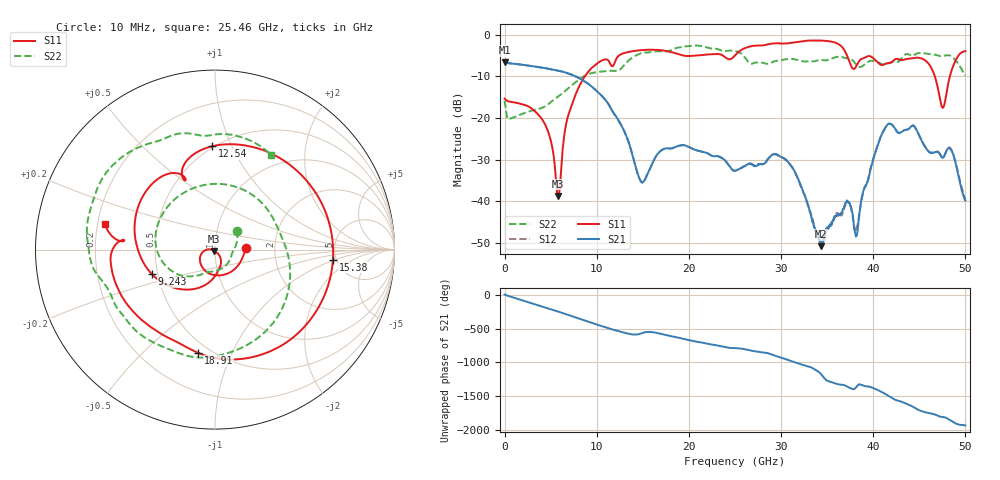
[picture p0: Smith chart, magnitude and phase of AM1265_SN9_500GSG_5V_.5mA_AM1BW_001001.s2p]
!Keysight Technologies,N5245B,MY58422270,A.16.20.02
!Date: Thursday, March 05, 2026 00:32:22
!Correction: S11(C  2-Port  )
!S21(C  2-Port  )
!S12(C  2-Port  )
!S22(C  2-Port  )
!S2P File: Measurements: S11, S21, S12, S22:
# Hz S  dB  R 50
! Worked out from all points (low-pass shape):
!   3201 points, 10 MHz to 50 GHz, reference 50 ohm
!   highest |S21| = -6.62 dB at 10 MHz (marker M1); lowest = -50.7 dB at 34.36 GHz (marker M2)
!   |S21| within 3 dB of the highest: start of sweep to 7.338 GHz
!   lowest |S11| = -38.7 dB at 5.821 GHz (marker M3), VSWR 1.02, Z = 49.4 - j0.975 ohm
!   |S11| at or under -10 dB: start of sweep to 8.715 GHz; 46.69 GHz to 48.31 GHz (1.624 GHz wide, 3.42 % of centre)
!   |S22| runs from -20.3 to -2.6 dB; largest |S21 - S12| = 0.002
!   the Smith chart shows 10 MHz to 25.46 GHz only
!   S11 on the Smith chart (normalised r, x): 10 MHz: 1.41, +0.03; 9.243 GHz: 0.46, -0.15; 12.54 GHz: 0.49, +0.84; 15.38 GHz: 4.68, -0.93; 18.91 GHz: 0.43, -0.75; 25.46 GHz: 0.23, +0.11
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1e7  -15.34 3.3  -6.62 2.8  -6.65 3.0  -15.82 40.3
2.306416e9  -16.94 -91.6  -7.30 -97.9  -7.30 -97.9  -18.69 -83.1
4.649697e9  -22.77 -167.1  -8.11 162.3  -8.11 162.3  -16.82 -114.4
5.821338e9  -38.67 -122.1  -8.62 111.1  -8.61 111.2  -14.80 -126.6
6.743028e9  -20.80 -70.1  -9.16 69.5  -9.15 69.5  -13.18 -137.0
8.352081e9  -11.32 -124.8  -10.73 -4.6  -10.72 -4.6  -10.33 -168.9
9.242528e9  -8.47 -158.7  -12.03 -45.7  -12.02 -45.6  -9.32 165.2
1.253874e10  -4.79 91.7  -21.19 175.4  -21.21 175.5  -8.33 7.4
1.538192e10  -3.62 -4.9  -34.04 168.8  -34.02 168.9  -4.28 -112.0
1.667854e10  -3.65 -43.5  -28.40 150.5  -28.40 150.7  -4.02 -142.2
1.891247e10  -4.68 -99.2  -26.65 84.5  -26.62 84.9  -3.07 -179.3
2.5005e10  -4.96 173.5  -32.67 -68.3  -32.58 -68.9  -3.91 71.2
2.545803e10  -4.00 166.9  -32.23 -73.9  -32.21 -73.9  -4.24 59.6
3.039455e10  -2.11 82.1  -29.77 133.2  -29.89 133.1  -5.92 -46.2
3.334708e10  -1.39 35.5  -44.21 0.4  -43.73 4.5  -6.39 -127.8
3.43625e10  -1.39 17.9  -50.72 -97.6  -50.31 -105.6  -6.05 -149.4
3.717444e10  -5.07 -41.1  -39.93 82.6  -40.08 83.7  -5.68 156.4
3.818986e10  -7.43 -22.4  -48.11 79.5  -46.62 74.7  -7.25 139.2
4.167354e10  -6.81 -54.5  -21.37 -57.2  -21.36 -57.5  -6.82 114.0
4.509473e10  -5.59 -102.3  -24.67 87.6  -24.65 88.6  -4.37 75.1
4.770358e10  -16.86 70.6  -29.17 -9.9  -29.02 -9.6  -5.04 40.8
5e10  -3.93 -73.2  -39.76 -132.1  -39.50 -127.0  -9.81 4.8
